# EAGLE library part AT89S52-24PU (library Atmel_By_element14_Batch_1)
8-bit Microcontroller
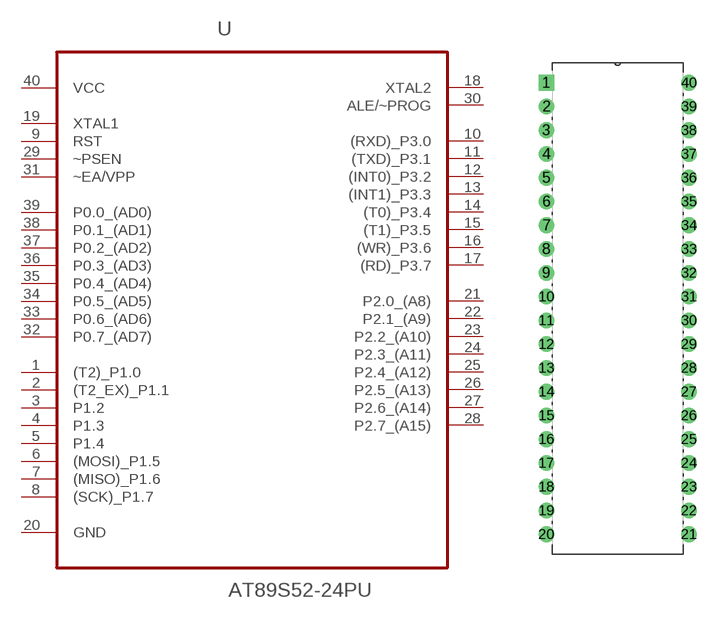
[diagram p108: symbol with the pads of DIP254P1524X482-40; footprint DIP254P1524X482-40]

Designator prefix U

## AT89S52-24PU (DESCRIPTION: 8-bit Microcontroller; MPN: AT89S52-24PU; OC_FARNELL: 1095743; OC_NEWARK: 96K6580; PACKAGE: DIP-40; SUPPLIER: Atmel)  [DIP254P1524X482-40]
1  (T2)_P1.0
2  (T2_EX)_P1.1
3  P1.2
4  P1.3
5  P1.4
6  (MOSI)_P1.5
7  (MISO)_P1.6
8  (SCK)_P1.7
9  RST  in
10  (RXD)_P3.0
11  (TXD)_P3.1
12  (INT0)_P3.2
13  (INT1)_P3.3
14  (T0)_P3.4
15  (T1)_P3.5
16  (WR)_P3.6
17  (RD)_P3.7
18  XTAL2  out
19  XTAL1  in
20  GND  pas
21  P2.0_(A8)
22  P2.1_(A9)
23  P2.2_(A10)
24  P2.3_(A11)
25  P2.4_(A12)
26  P2.5_(A13)
27  P2.6_(A14)
28  P2.7_(A15)
29  ~PSEN  in
30  ALE/~PROG  out
31  ~EA/VPP  in
32  P0.7_(AD7)
33  P0.6_(AD6)
34  P0.5_(AD5)
35  P0.4_(AD4)
36  P0.3_(AD3)
37  P0.2_(AD2)
38  P0.1_(AD1)
39  P0.0_(AD0)
40  VCC  pwr

## Footprint DIP254P1524X482-40 (pad centres in mm)
drill 1.118 square: 1 -15.24,48.26
drill 1.118: 2 -15.24,45.72; 3 -15.24,43.18; 4 -15.24,40.64; 5 -15.24,38.1; 6 -15.24,35.56; 7 -15.24,33.02; 8 -15.24,30.48; 9 -15.24,27.94; 10 -15.24,25.4; 11 -15.24,22.86; 12 -15.24,20.32; 13 -15.24,17.78; 14 -15.24,15.24; 15 -15.24,12.7; 16 -15.24,10.16; 17 -15.24,7.62; 18 -15.24,5.08; 19 -15.24,2.54; 20 -15.24,0; 21 0,0; 22 0,2.54; 23 0,5.08; 24 0,7.62; 25 0,10.16; 26 0,12.7; 27 0,15.24; 28 0,17.78; 29 0,20.32; 30 0,22.86; 31 0,25.4; 32 0,27.94; 33 0,30.48; 34 0,33.02; 35 0,35.56; 36 0,38.1; 37 0,40.64; 38 0,43.18; 39 0,45.72; 40 0,48.26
